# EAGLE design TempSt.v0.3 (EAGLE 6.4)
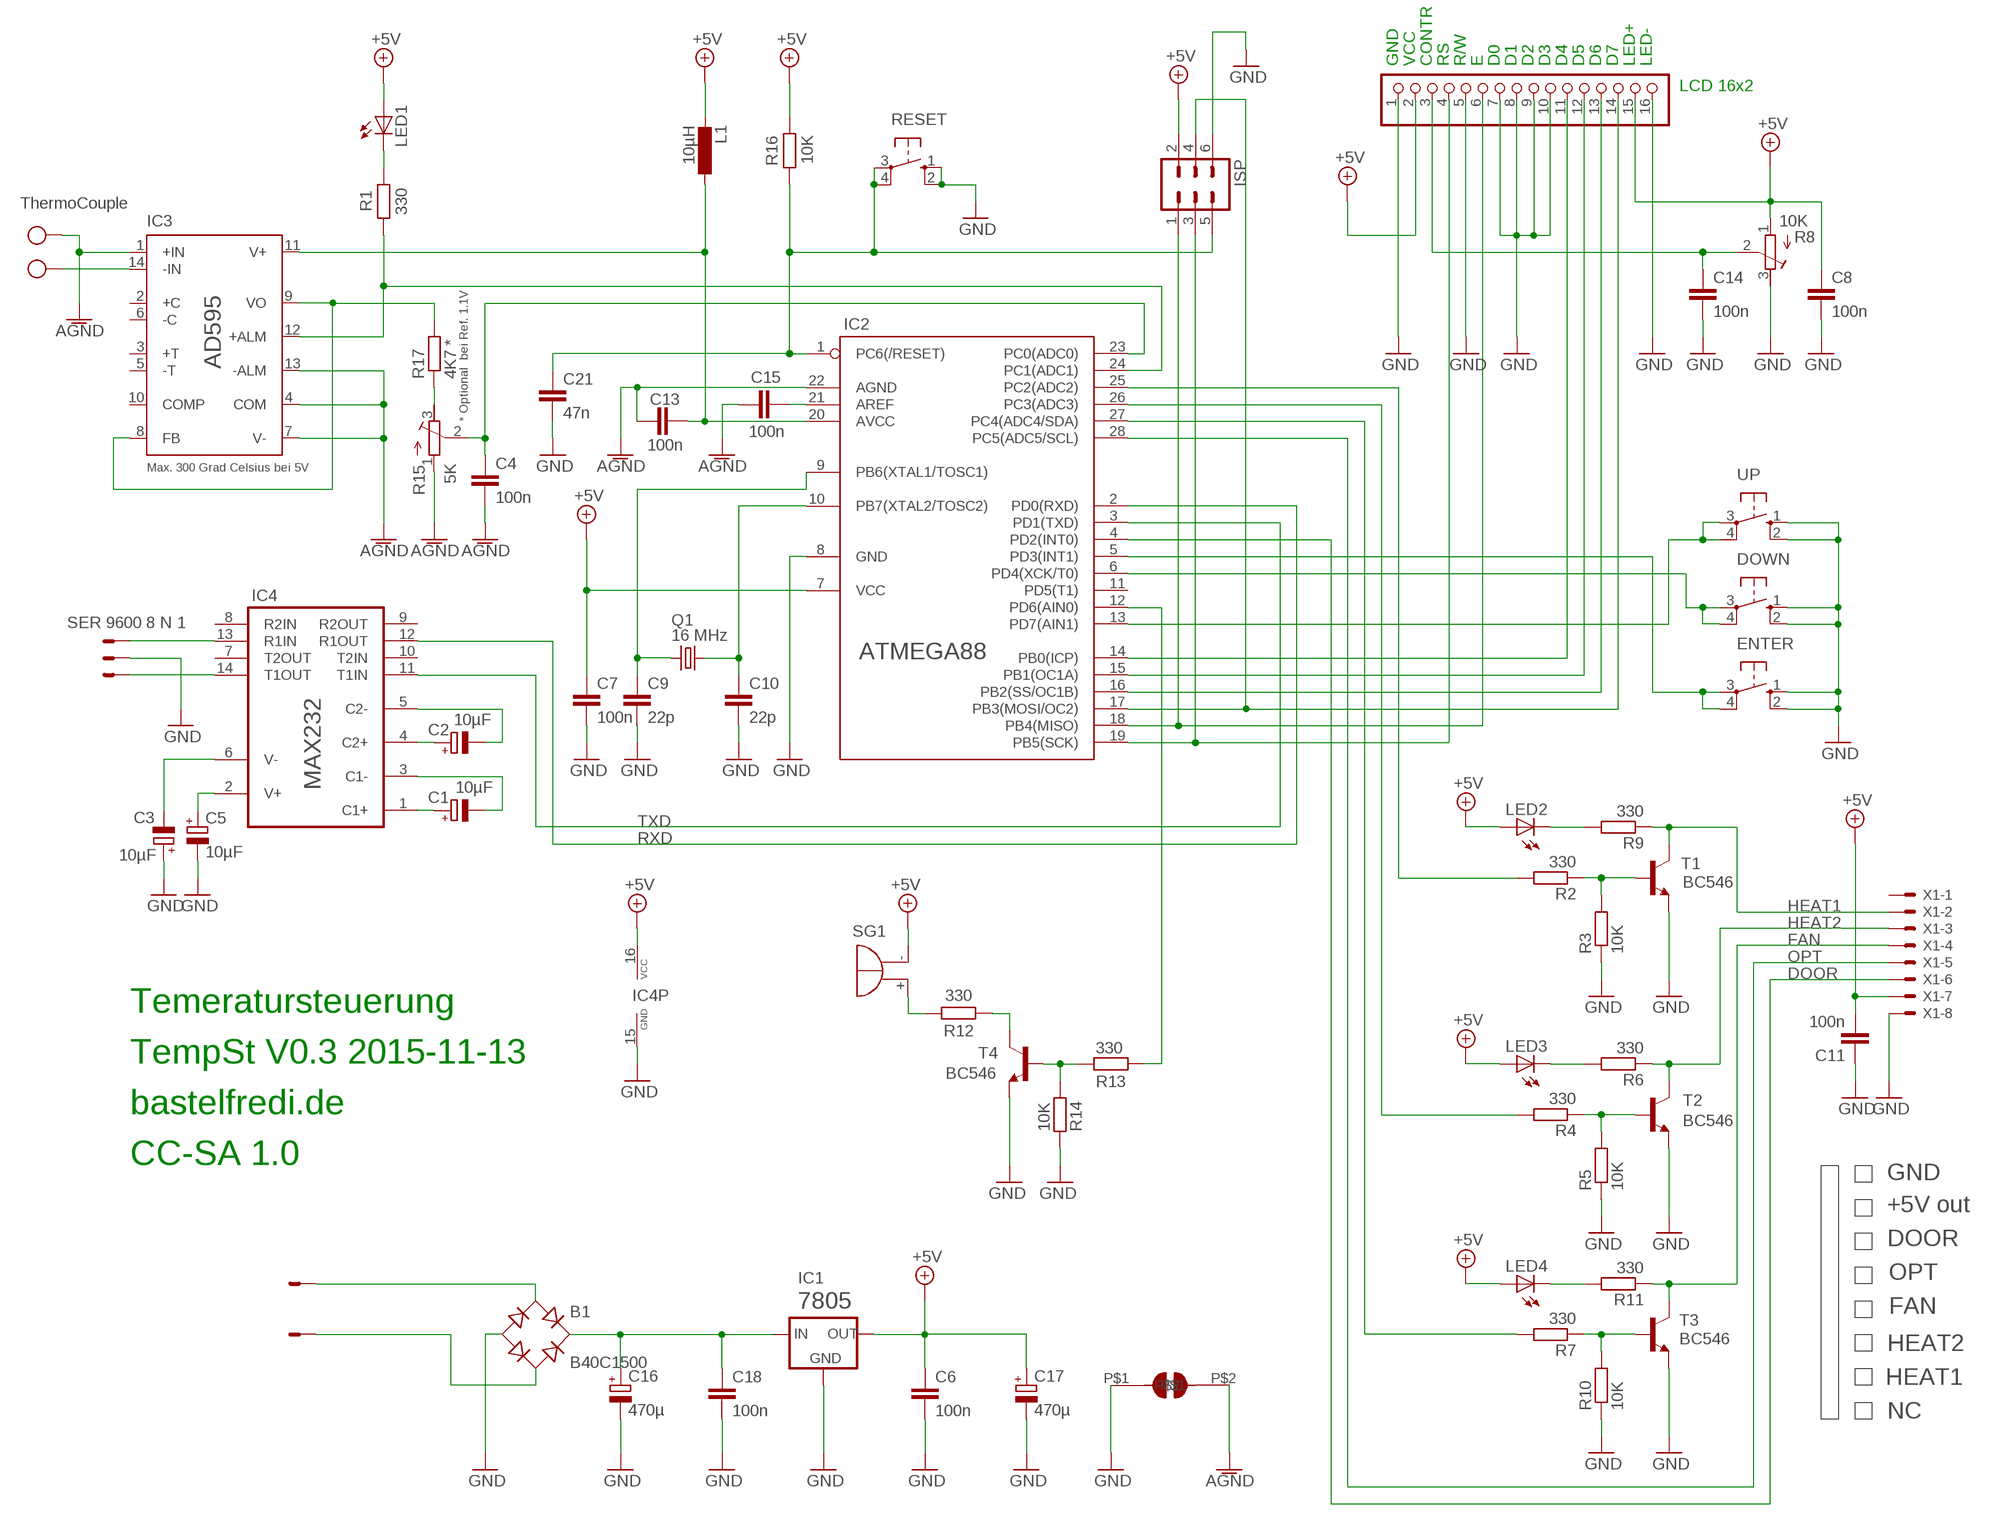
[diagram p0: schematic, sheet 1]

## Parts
B1  B40C1500  RB1A  [RB1A]
C1  10µF  CPOL-EUE2.5-6  [E2,5-6]
C2  10µF  CPOL-EUE2.5-6  [E2,5-6]
C3  10µF  CPOL-EUE2.5-6  [E2,5-6]
C4  100n  C-EU025-025X050  [C025-025X050]
C5  10µF  CPOL-EUE2.5-6  [E2,5-6]
C6  100n  C-EU050-035X075  [C050-035X075]
C7  100n  C-EU025-025X050  [C025-025X050]
C8  100n  C-EU025-025X050  [C025-025X050]
C9  22p  C-EU025-025X050  [C025-025X050]
C10  22p  C-EU025-025X050  [C025-025X050]
C11  100n  C-EU025-025X050  [C025-025X050]
C13  100n  C-EU025-025X050  [C025-025X050]
C14  100n  C-EU025-025X050  [C025-025X050]
C15  100n  C-EU025-025X050  [C025-025X050]
C16  470µ  CPOL-EUE5-10.5  [E5-10,5]
C17  470µ  CPOL-EUE5-10.5  [E5-10,5]
C18  100n  C-EU050-035X075  [C050-035X075]
C21  47n  C-EU050-025X075  [C050-025X075]
DOWN  10-XX  [B3F-10XX]
ENTER  10-XX  [B3F-10XX]
IC1  7805  78XXL  [78XXL]
IC2  ATMEGA88  MEGA8-P  [DIL28-3]
IC3  AD595  [DIL14]
IC4  MAX232  [DIL16]
ISP  ML6  [ML6]
JP3  LCD  PINHD-1X16  [1X16]
L1  10µH  L-EU0207/10  [0207/10]
LED1  LED3MM  [LED3MM]
LED2  LED3MM  [LED3MM]
LED3  LED3MM  [LED3MM]
LED4  LED3MM  [LED3MM]
Q1  16 MHz  CRYSTALHC49U-V  [HC49U-V]
R1  330  R-EU_0207/7  [0207/7]
R2  330  R-EU_0207/7  [0207/7]
R3  10K  R-EU_0207/7  [0207/7]
R4  330  R-EU_0207/7  [0207/7]
R5  10K  R-EU_0207/7  [0207/7]
R6  330  R-EU_0207/7  [0207/7]
R7  330  R-EU_0207/7  [0207/7]
R8  10K  R-TRIMM3339P  [RTRIM3339P]
R9  330  R-EU_0207/7  [0207/7]
R10  10K  R-EU_0207/7  [0207/7]
R11  330  R-EU_0207/7  [0207/7]
R12  330  R-EU_0207/7  [0207/7]
R13  330  R-EU_0207/7  [0207/7]
R14  10K  R-EU_0207/7  [0207/7]
R15  5K  R-TRIMM64W  [RTRIM64W]
R16  10K  R-EU_0207/7  [0207/7]
R17  4K7 *  R-EU_0207/10  [0207/10]
RESET  10-XX  [B3F-10XX]
SER  SER 9600 8 N 1  22-23-2031  [22-23-2031]
SG1  F/QMBIII  [F/QMBIII]
T1  BC546  BC548-NPN-TO92-CBE  [TO92-CBE]
T2  BC546  BC548-NPN-TO92-CBE  [TO92-CBE]
T3  BC546  BC548-NPN-TO92-CBE  [TO92-CBE]
T4  BC546  BC548-NPN-TO92-CBE  [TO92-CBE]
TC  ThermoCouple  AK500/2  [AK500/2]
U$1  SOLDER_JUMPER  [SOLDER_JUMPER]
UP  10-XX  [B3F-10XX]
X1  22-23-2081  [22-23-2081]
X4  22-23-2021  [22-23-2021]

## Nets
+5V: C6.1 C7.1 C8.1 C11.2 C17.+ IC1.OUT IC2.7(VCC) IC4.16(VCC) ISP.2 JP3.2 JP3.15 L1.2 LED1.A LED2.A LED3.A LED4.A R8.1(E) R16.2 SG1.-(+) X1.7
AGND: C4.2 C13.1 C15.2 IC2.22(AGND) IC3.1(+IN) IC3.4(COM) IC3.7(V-) IC3.13(-ALM) R15.1(E) TC.2 U$1.P$2
DOOR: IC2.4(PD2(INT0)) X1.6
ENTER: DOWN.3(P) DOWN.4(P1) IC2.6(PD4(XCK/T0))
FAN: R11.1 T3.C X1.4
GND: B1.- C3.+ C5.- C6.2 C7.2 C8.2 C9.2 C10.2 C11.1 C14.2 C16.- C17.- C18.2 C21.2 DOWN.1(S) DOWN.2(S1) ENTER.1(S) ENTER.2(S1) IC1.GND IC2.8(GND) IC4.15(GND) ISP.6 JP3.1 JP3.5 JP3.7 JP3.8 JP3.9 JP3.10 JP3.16 R3.1 R5.1 R8.3(A) R10.1 R14.1 RESET.1(S) RESET.2(S1) SER.2 T1.E T2.E T3.E T4.E U$1.P$1 UP.1(S) UP.2(S1) X1.8
HEAT1: R9.1 T1.C X1.2
HEAT2: R6.1 T2.C X1.3
N$1: IC4.14(T1OUT) SER.1
N$2: IC2.13(PD7(AIN1)) UP.3(P) UP.4(P1)
N$3: C15.1 IC2.21(AREF)
N$4: IC3.8(FB) IC3.9(VO) R17.2
N$5: IC2.17(PB3(MOSI/OC2)) ISP.4 JP3.14
N$6: IC2.18(PB4(MISO)) ISP.1 JP3.6
N$8: R12.1 SG1.+(-)
N$9: IC2.19(PB5(SCK)) ISP.3 JP3.4
N$10: LED1.K(C) R1.2
N$11: IC2.14(PB0(ICP)) JP3.11
N$12: IC2.15(PB1(OC1A)) JP3.12
N$13: IC2.16(PB2(SS/OC1B)) JP3.13
N$14: C14.1 JP3.3 R8.2(S)
N$15: IC2.24(PC1(ADC1)) IC3.12(+ALM) R1.1
N$16: B1.AC2 X4.1
N$17: B1.+ C16.+ C18.1 IC1.IN
N$18: IC4.13(R1IN) SER.3
N$20: LED2.K(C) R9.2
N$21: C5.+ IC4.2(V+)
N$22: C3.- IC4.6(V-)
N$23: C2.- IC4.5(C2-)
N$24: C1.- IC4.3(C1-)
N$25: C10.1 IC2.10(PB7(XTAL2/TOSC2)) Q1.2
N$26: C9.1 IC2.9(PB6(XTAL1/TOSC1)) Q1.1
N$27: C1.+ IC4.1(C1+)
N$28: C2.+ IC4.4(C2+)
N$29: R15.3(A) R17.1
N$30: R2.1 R3.2 T1.B
N$31: C21.1 IC2.1(PC6(/RESET)) ISP.5 R16.1 RESET.3(P) RESET.4(P1)
N$32: LED3.K(C) R6.2
N$33: IC2.25(PC2(ADC2)) R2.2
N$34: C4.1 IC2.23(PC0(ADC0)) R15.2(S)
N$35: R4.1 R5.2 T2.B
N$36: IC2.26(PC3(ADC3)) R4.2
N$37: LED4.K(C) R11.2
N$38: C13.2 IC2.20(AVCC) IC3.11(V+) L1.1
N$39: R7.1 R10.2 T3.B
N$40: IC2.27(PC4(ADC4/SDA)) R7.2
N$41: R12.2 T4.C
N$43: IC3.14(-IN) TC.1
N$46: R13.1 R14.2 T4.B
N$47: ENTER.3(P) ENTER.4(P1) IC2.5(PD3(INT1))
N$48: IC2.12(PD6(AIN0)) R13.2
N$49: B1.AC1 X4.2
OPT: IC2.28(PC5(ADC5/SCL)) X1.5
RXD: IC2.2(PD0(RXD)) IC4.12(R1OUT)
TXD: IC2.3(PD1(TXD)) IC4.11(T1IN)
Unconnected: IC2.11(PD5(T1)) IC3.2(+C) IC3.3(+T) IC3.5(-T) IC3.6(-C) IC3.10(COMP) IC4.7(T2OUT) IC4.8(R2IN) IC4.9(R2OUT) IC4.10(T2IN) X1.1

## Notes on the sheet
- GND | VCC | CONTR | RS | R/W | E | D0 | D1 | D2 | D3 | D4 | D5 | D6 | D7 | LED+ | LED-
- LCD 16x2
- * Optional  bei Ref. 1.1V
- Max. 300 Grad Celsius bei 5V
- Temeratursteuerung
- TempSt V0.3 2015-11-13
- bastelfredi.de
- CC-SA 1.0
- GND
- +5V out
- DOOR
- OPT
- FAN
- HEAT2
- HEAT1
- NC

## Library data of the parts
B1 = rectifier:RB1A: RECTIFIER 1 A
C1-C3 C5 C16 C17 = rcl:CPOL-EU: POLARIZED CAPACITOR, European symbol
C4 C6-C11 C13-C15 C18 C21 = rcl:C-EU: CAPACITOR, European symbol
DOWN ENTER RESET UP = buttons:10-XX: OMRON SWITCH
IC1 = v-reg:78XXL: VOLTAGE REGULATOR
IC2 = atmel:MEGA8-P: MICROCONTROLLER 8 Kbytes FLASH, 1 kbytes SRAM, 512 bytes EEPROM, USART, 4-channel 10 bit ADC, 2-channel 8 bit ADC Pin compatible with Atmega48, ATMega88, ATMega168 Source: avr.lbr
IC3 = analog-devices:AD595: ANALOG DEVICES; MPN: AD595AQ; OC_FARNELL: 409194; OC_NEWARK: 06WX1596
IC4 = maxim:MAX232: RS232 TRANSEIVER; MF: MAXIM; MPN: MAX232ACPE+; OC_FARNELL: 9723773; OC_NEWARK: 68K4544
ISP = con-harting-ml:ML6: HARTING; OC_FARNELL: unknown; OC_NEWARK: unknown
JP3 = pinhead:PINHD-1X16: PIN HEADER
L1 = rcl:L-EU: INDUCTOR, European symbol
LED1-LED4 = led:LED: LED
Q1 = crystal:CRYSTAL: CRYSTAL
R1-R7 R9-R14 R16 R17 = rcl:R-EU_: RESISTOR, European symbol
R8 R15 = rcl:R-TRIMM: Trimm resistor
SER = con-molex:22-23-2031: .100" (2.54mm) Center Header - 3 Pin; MF: MOLEX; MPN: 22-23-2031; OC_FARNELL: 1462950; OC_NEWARK: 30C0862
SG1 = buzzer:F/QMBIII: BUZZER; OC_FARNELL: unknown; OC_NEWARK: unknown
T1-T4 = transistor:*-NPN-: NPN Transistror BF959 corrected 2008.03.06
TC = con-ptr500:AK500/2: CONNECTOR; OC_FARNELL: unknown; OC_NEWARK: unknown
U$1 = th:SOLDER_JUMPER
X1 = con-molex:22-23-2081: .100" (2.54mm) Center Header - 8 Pin; MF: MOLEX; MPN: 22-23-2081; OC_FARNELL: 1756826; OC_NEWARK: 01C7592
X4 = con-molex:22-23-2021: .100" (2.54mm) Center Header - 2 Pin; MF: MOLEX; MPN: 22-23-2021; OC_FARNELL: 1462926; OC_NEWARK: 25C3832

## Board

Size 92.38 x 83.82 mm. Coordinates in mm from the lower left corner, seen from the top.
Outline: 0,83.81 92.38,83.81 92.38,0 0,0 0,83.82
Copper layers (1*16): Top 0.035mm / dielectric 1.5mm / Bottom 0.035mm
Design rules "default": minimum track width 10mil, minimum drill 24mil, track to track 8mil, track to pad 8mil, pad to pad 8mil, via to via 8mil, smd to smd 8mil, copper to edge 40mil, drill to drill 8mil, minimum pad ring 10mil, minimum via ring 8mil, stop-mask expansion 4mil, vias tented up to drill 0mil, thermal gap 10mil

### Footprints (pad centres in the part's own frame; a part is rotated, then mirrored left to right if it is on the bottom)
RB1A = drill 1.016: + -2.54,2.54 | drill 1.016 octagon: - 2.54,-2.54; AC1 2.54,2.54; AC2 -2.54,-2.54
E2,5-6 = drill 0.813 pad 1.6: + -1.27,0 | drill 0.813 pad 1.6 octagon: - 1.27,0
C025-025X050 = drill 0.813 octagon: 1 -1.27,0; 2 1.27,0
C050-035X075 = drill 0.813 octagon: 1 -2.54,0; 2 2.54,0
E5-10,5 = drill 1.016 pad 2.54: + -2.54,0 | drill 1.016 pad 2.54 octagon: - 2.54,0
C050-025X075 = drill 0.813 octagon: 1 -2.54,0; 2 2.54,0
B3F-10XX = drill 1.016 long: 1 -3.251,2.261; 2 3.251,2.261; 3 -3.251,-2.261; 4 3.251,-2.261
78XXL = drill 1.016 long: GND 0,-3.81; IN -2.54,-3.81; OUT 2.54,-3.81 | hole 3.302: 0,11.176
DIL28-3 = drill 0.813 long: 1 -16.51,-3.81; 2 -13.97,-3.81; 3 -11.43,-3.81; 4 -8.89,-3.81; 5 -6.35,-3.81; 6 -3.81,-3.81; 7 -1.27,-3.81; 8 1.27,-3.81; 9 3.81,-3.81; 10 6.35,-3.81; 11 8.89,-3.81; 12 11.43,-3.81; 13 13.97,-3.81; 14 16.51,-3.81; 15 16.51,3.81; 16 13.97,3.81; 17 11.43,3.81; 18 8.89,3.81; 19 6.35,3.81; 20 3.81,3.81; 21 1.27,3.81; 22 -1.27,3.81; 23 -3.81,3.81; 24 -6.35,3.81; 25 -8.89,3.81; 26 -11.43,3.81; 27 -13.97,3.81; 28 -16.51,3.81
DIL14 = drill 0.813 long: 1 -7.62,-3.81; 2 -5.08,-3.81; 3 -2.54,-3.81; 4 0,-3.81; 5 2.54,-3.81; 6 5.08,-3.81; 7 7.62,-3.81; 8 7.62,3.81; 9 5.08,3.81; 10 2.54,3.81; 11 0,3.81; 12 -2.54,3.81; 13 -5.08,3.81; 14 -7.62,3.81
DIL16 = drill 0.813 long: 1 -8.89,-3.81; 2 -6.35,-3.81; 3 -3.81,-3.81; 4 -1.27,-3.81; 5 1.27,-3.81; 6 3.81,-3.81; 7 6.35,-3.81; 8 8.89,-3.81; 9 8.89,3.81; 10 6.35,3.81; 11 3.81,3.81; 12 1.27,3.81; 13 -1.27,3.81; 14 -3.81,3.81; 15 -6.35,3.81; 16 -8.89,3.81
ML6 = drill 0.914 octagon: 1 -2.54,-1.27; 2 -2.54,1.27; 3 0,-1.27; 4 0,1.27; 5 2.54,-1.27; 6 2.54,1.27
1X16 = drill 1.016 long: 1 -19.05,0; 2 -16.51,0; 3 -13.97,0; 4 -11.43,0; 5 -8.89,0; 6 -6.35,0; 7 -3.81,0; 8 -1.27,0; 9 1.27,0; 10 3.81,0; 11 6.35,0; 12 8.89,0; 13 11.43,0; 14 13.97,0; 15 16.51,0; 16 19.05,0
0207/10 = drill 0.813 octagon: 1 -5.08,0; 2 5.08,0
LED3MM = drill 0.813 octagon: A -1.27,0; K 1.27,0
HC49U-V = drill 0.813: 1 -2.413,0; 2 2.413,0
0207/7 = drill 0.813 octagon: 1 -3.81,0; 2 3.81,0
RTRIM3339P = drill 0.61: 1 -2.54,0; 2 0,-2.54; 3 2.54,0
RTRIM64W = drill 0.61: 1 1.27,-2.54; 2 1.27,0; 3 1.27,2.54
22-23-2031 = drill 1 long: 1 -2.54,0; 2 0,0; 3 2.54,0
F/QMBIII = drill 0.914 pad 2.159 octagon: + 3.251,0; - -3.251,0
TO92-CBE = drill 0.813 long: B 0,0; C -2.54,0; E 2.54,0
AK500/2 = drill 1.321 long: 1 -2.515,0; 2 2.515,0
SOLDER_JUMPER = drill 0.8 square: P$1 -1.905,0; P$2 1.905,0
22-23-2081 = drill 1 long: 1 -8.89,0; 2 -6.35,0; 3 -3.81,0; 4 -1.27,0; 5 1.27,0; 6 3.81,0; 7 6.35,0; 8 8.89,0
22-23-2021 = drill 1 long: 1 -1.27,0; 2 1.27,0

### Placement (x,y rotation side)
B1  19.05,15.24 90 top
C1  87.63,16.51 90 top
C2  87.63,22.86 90 top
C3  87.63,29.21 270 top
C4  58.42,42.55 180 top
C5  87.63,10.16 270 top
C6  10.15,19.07 180 top
C7  59.69,62.23 180 top
C8  53.34,76.2 90 top
C9  53.34,60.96 270 top
C10  48.26,60.96 270 top
C11  71.12,11.43 90 top
C13  27.94,13.34 90 top
C14  6.35,73.66 180 top
C15  54.61,39.37 270 top
C16  11.43,7.62 90 top
C17  20.32,26.67 90 top
C18  7.62,15.24 0 top
C21  77.47,57.15 90 top
DOWN  87.63,60.96 270 top
ENTER  87.63,49.53 270 top
IC1  8.89,27.94 0 top
IC2  55.88,49.52 180 top
IC3  35.56,19.05 90 top
IC4  78.74,20.32 90 top
ISP  26.67,38.1 180 top
JP3  29.21,77.47 0 top
L1  27.94,22.23 90 top
LED1  45.72,8.89 180 top
LED2  45.72,31.75 0 top
LED3  45.72,24.13 0 top
LED4  45.72,16.51 0 top
Q1  50.8,66.04 180 top
R1  38.1,31.11 0 top
R2  60.96,33.02 0 top
R3  52.07,34.29 0 top
R4  60.96,25.4 0 top
R5  52.07,26.67 0 top
R6  52.07,22.86 180 top
R7  60.96,17.78 0 top
R8  7.62,67.31 270 top
R9  52.07,30.48 180 top
R10  52.07,19.05 0 top
R11  52.07,15.24 180 top
R12  71.12,67.31 180 top
R13  71.12,72.39 180 top
R14  71.12,76.2 180 top
R15  60.96,38.1 270 top
R16  73.66,59.69 90 top
R17  40.64,35.56 180 top
RESET  87.63,38.1 270 top
SER  80.01,5.08 0 top
SG1  76.2,37.47 0 top
T1  60.96,29.21 0 top
T2  60.96,21.59 0 top
T3  60.96,13.97 0 top
T4  78.74,72.39 90 top
TC  35.56,5.08 0 top
U$1  27.94,6.35 90 top
UP  87.63,72.39 270 top
X1  60.96,5.08 0 top
X4  21.59,5.08 0 top

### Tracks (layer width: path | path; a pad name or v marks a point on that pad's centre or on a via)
+5V  (via drill 0.6 pad 1.42)
  Top 1.016: v39.37,68.58 v17.78,68.58 | v17.78,64.77 v17.78,33.02
  Top 1.27: v44.45,29.21 v27.94,29.21 | v48.26,10.16 v68.58,10.16 | v60.96,64.77 v60.96,74.93
  Bottom 0.61: IC2.7
  Bottom 1.016: SG1.- 72.39,36.91 72.39,20.32 69.85,17.78 69.85,12.7 | IC4.16 73.66,11.43 72.39,12.7 C11.2 69.85,12.7 | 69.85,12.7 69.85,11.43 v68.58,10.16
  Bottom 1.27: X1.7 67.31,8.89 v68.58,10.16
  Bottom 1.778: R16.2 60.96,63.5 | 60.96,63.5 C7.1 60.96,58.42 57.15,54.61 IC2.7 | 12.7,69.85 16.51,69.85 v17.78,68.58 v17.78,64.77 | IC2.7 | LED2.A v44.45,29.21 LED3.A LED4.A 44.45,12.7 46.99,10.16 | L1.2 27.94,27.94 | 27.94,27.94 v27.94,29.21 | v27.94,29.21 27.94,31.75 | 27.94,31.75 27.94,33.02 | 27.94,33.02 27.94,34.29 29.21,35.56 ISP.2 | 12.7,69.85 R8.1 | JP3.15 45.72,73.66 | 45.72,73.66 44.45,73.66 v39.37,68.58 | 45.72,73.66 52.07,73.66 C8.1 v60.96,74.93 | v48.26,10.16 46.99,10.16 | 46.99,10.16 LED1.A | 60.96,63.5 v60.96,64.77 | JP3.2 12.7,69.85 | IC1.OUT 12.7,24.13 | C6.1 11.43,20.32 IC1.OUT | IC1.OUT C17.+ 24.13,24.13 26.67,26.67 | 26.67,26.67 27.94,27.94 | v17.78,33.02 24.13,33.02 | 24.13,33.02 25.4,31.75 | 25.4,31.75 26.67,30.48 | 26.67,30.48 v27.94,29.21 | 24.13,33.02 27.94,33.02 | 25.4,31.75 27.94,31.75 | 26.67,30.48 26.67,26.67
AGND  (1 unrouted)
  Bottom 0.61: 35.56,13.97 38.1,11.43
  Bottom 1.27: 36.83,19.05 36.83,15.24 35.56,13.97 IC3.13 | IC3.4 36.83,19.05 | 36.83,19.05 36.83,26.04 37.47,26.67 IC3.7 39.37,31.75 40.64,33.02 41.91,33.02 43.18,34.29 43.18,36.83 44.45,38.1 C15.2 57.15,38.1 | 57.15,41.91 IC2.22 | 57.15,41.91 57.15,39.37 57.15,38.1 | 30.48,13.97 28.57,12.06 C13.1 U$1.P$2 | 57.15,41.91 C4.2 | R15.1 57.15,38.1
  Bottom 1.778: IC3.1 39.37,6.38 TC.2 | IC3.1 38.1,10.16 38.1,5.08 36.83,6.35 | 36.83,6.35 36.83,10.16 38.1,11.43 IC3.1 | 36.83,6.35 36.83,5.08 38.1,3.81 39.37,5.08 39.37,6.35
DOOR
  Bottom 0.61: IC2.4 64.77,50.8 67.31,48.26 73.66,48.26 74.3,47.62 74.3,43.81 70.48,40.01 70.48,20.95 68.58,19.05 68.58,13.34 64.77,9.53 X1.6
ENTER
  Bottom 0.61: IC2.6 59.69,54.61 62.23,57.15 64.77,57.15 68.58,60.96 74.93,60.96 76.2,62.23 80.01,62.23 85.09,57.15 85.37,57.43 DOWN.4 DOWN.3
FAN
  Bottom 0.61: X1.4 59.69,10.16 58.42,11.43 T3.C 57.15,15.24 R11.1
GND  (via drill 0.6 pad 1.42, 0.8, 2)  (1 unrouted)
  Top 1.27: v58.42,78.74 v58.42,67.31 | v65.41,15.24 v71.75,15.24
  Bottom 0.61: 50.8,59.69 50.8,51.44 51.44,50.8 53.98,50.8 54.61,51.43 IC2.8 | R14.1 77.47,76.2 T4.E
  Bottom 1.016: C9.2 50.8,59.69 | 50.8,59.69 C10.2 | 57.15,62.23 57.15,57.78 54.61,55.24 IC2.8 | C21.2 79.38,59.69 83.82,55.24 89.89,55.24 | 50.8,59.69 50.8,67.31 52.07,68.58 55.88,68.58 57.15,67.31 57.15,62.23 | 57.15,62.23 C7.2 | 71.12,8.89 76.2,8.89 77.47,10.16 77.47,12.7 76.2,13.97 IC4.15 73.66,13.97 72.39,15.24 v71.75,15.24 | C3.+ 89.53,30.48 90.81,29.21 90.81,10.16 89.53,8.89 C5.- | T4.E 81.28,74.93 82.55,73.66 82.55,67.31 83.19,66.67 89.89,66.67 | X1.8 71.12,6.35 71.12,8.89 | 71.12,8.89 C11.1
  Bottom 1.27: JP3.7 25.4,81.28 | T3.E 63.5,15.24 | 63.5,15.24 62.23,16.51 62.23,19.05 63.5,20.32 T2.E 63.5,22.86 62.23,24.13 62.23,26.67 63.5,27.94 T1.E | R3.1 49.53,34.29 50.8,33.02 50.8,26.67 | R5.1 50.8,26.67 | 50.8,26.67 50.8,21.59 R10.1 50.8,16.51 50.8,8.26 49.53,6.99 49.53,1.27 | X1.8 69.85,1.27 | SER.2 80.01,1.27 | 33.02,81.28 JP3.10 | JP3.5 20.32,81.28 | JP3.8 27.94,81.28 | JP3.9 30.48,81.28 | 57.15,67.31 v58.42,67.31 | U$1.P$1 27.94,1.27 | v65.41,15.24 63.5,15.24
  Bottom 1.778: 48.26,81.28 33.02,81.28 30.48,81.28 27.94,81.28 25.4,81.28 20.32,81.28 11.43,81.28 10.16,80.01 JP3.1 6.35,77.47 2.54,73.66 | 48.26,81.28 JP3.16 C8.2 | v45.09,1.27 27.94,1.27 10.16,1.27 2.54,8.89 2.54,27.94 | v45.09,1.27 49.53,1.27 69.85,1.27 80.01,1.27 83.82,1.27 85.09,2.54 85.09,6.35 C5.- | 2.54,29.21 2.54,41.91 6.35,41.91 | 6.35,41.91 8.89,41.91 | 8.89,41.91 8.89,43.18 | 8.89,43.18 8.89,44.45 | 8.89,44.45 8.89,49.53 | 8.89,49.53 8.89,52.07 6.35,52.07 | 6.35,52.07 2.54,52.07 2.54,64.77 | 2.54,64.77 2.54,73.66 | 48.26,81.28 58.42,81.28 | 58.42,81.28 83.82,81.28 89.46,75.64 UP.1 UP.2 89.89,66.67 DOWN.1 DOWN.2 89.89,55.24 ENTER.1 ENTER.2 RESET.1 RESET.2 89.89,32.74 C3.+ | 2.54,64.77 R8.3 8.89,63.5 | C14.2 2.54,73.66 | 58.42,81.28 v58.42,78.74 | 8.89,27.94 10.16,29.21 13.97,29.21 | 8.89,27.94 IC1.GND 8.89,20.35 C6.2 10.16,16.51 C18.2 10.16,11.43 C16.- 12.7,11.43 12.7,12.7 15.24,15.24 19.05,15.24 B1.- | C17.- 15.24,29.21 | 15.24,29.21 13.97,29.21 | 2.54,27.94 2.54,29.21 | 2.54,29.21 3.81,29.21 | 3.81,29.21 7.62,29.21 8.89,27.94 | v45.09,5.08 v45.09,1.27 | ISP.6 15.24,36.83 | 15.24,36.83 13.97,36.83 | 13.97,36.83 13.97,35.56 | 13.97,35.56 13.97,30.48 | 13.97,30.48 13.97,29.21 | 8.89,41.91 13.97,41.91 13.97,38.1 | 13.97,38.1 13.97,36.83 | 6.35,52.07 8.89,49.53 | 6.35,41.91 8.89,44.45 | 8.89,43.18 11.43,43.18 11.43,41.91 12.7,40.64 12.7,36.83 10.16,34.29 8.89,34.29 5.08,38.1 5.08,40.64 11.43,40.64 11.43,36.83 10.16,35.56 8.89,35.56 6.35,38.1 6.35,39.37 10.16,39.37 10.16,38.1 | 10.16,38.1 10.16,36.83 8.89,36.83 7.62,38.1 10.16,38.1 | 15.24,36.83 13.97,35.56 | 15.24,29.21 13.97,30.48 | 15.24,36.83 13.97,38.1
  Bottom 1.778: 2.54,27.94 3.81,29.21
  other vias: 8.89,39.37
  pour Bottom (isolate 0.61): 44.45,69.22 56.52,69.22 58.42,67.31 58.42,55.88 57.15,54.61 46.99,54.61 44.45,57.15
  pour Bottom: 2.54,41.91 13.97,41.91 13.97,29.21 2.54,29.21
  pour Bottom: 8.89,41.91 13.97,41.91 13.97,57.15 13.97,58.42 7.62,64.77 2.54,64.77 2.54,52.07 8.89,52.07
HEAT1
  Bottom 0.61: T1.C 57.15,30.48 R9.1 53.34,27.94 53.34,21.59 52.7,20.95 52.7,12.06 54.61,10.16 X1.2
HEAT2
  Bottom 0.61: T2.C 57.15,22.86 R6.1 54.61,21.59 54.61,20.32 53.98,19.68 53.98,13.34 57.15,10.16 X1.3
N$1
  Bottom 0.61: SER.1 77.47,6.99 78.74,8.26 78.74,15.24 77.47,16.51 IC4.14
N$2
  Bottom 0.406: IC2.13
  Bottom 0.61: IC2.13 41.91,67.94 45.72,71.75 62.87,71.75 64.77,73.66 64.77,77.47 66.04,78.74 82.27,78.74 UP.3 UP.4
N$3
  Bottom 1.27: C15.1 IC2.21
N$4  (via drill 0.9 pad 1.68)
  Bottom 0.61: IC3.9 IC3.8 31.75,27.94 29.84,29.84 29.84,32.38 33.02,35.56 R17.2 v35.56,39.37
N$5  (via drill 0.6 pad 1.42)
  Top 0.61: v25.4,64.77 v39.37,64.77
  Bottom 0.406: IC2.17
  Bottom 0.61: JP3.14 43.18,76.2 36.83,69.85 36.83,67.31 v39.37,64.77 36.83,62.23 36.83,50.8 38.1,49.53 42.55,49.53 44.45,47.62 IC2.17 | ISP.4 27.94,38.1 27.94,43.18 25.4,45.72 v25.4,64.77
N$6  (via drill 0.6 pad 1.42)
  Top 0.61: v29.21,46.35 v33.66,46.35
  Bottom 0.61: IC2.18 46.99,44.45 45.72,43.18 36.83,43.18 v33.66,46.35 33.02,46.99 33.02,48.26 29.21,52.07 29.21,71.12 26.04,74.3 23.5,74.3 22.86,74.93 JP3.6 | ISP.1 v29.21,46.35
N$7  (via drill 2.2 pad 1.42)
  other vias: 90.17,81.28
N$8  (via drill 0.8 pad 1.42)
  Top 0.61: v83.19,62.23 v83.19,39.37
  Bottom 0.61: R12.1 78.11,67.31 v83.19,62.23 | v83.19,39.37 81.28,37.47 SG1.+
N$9
  Bottom 0.61: IC2.19 49.53,43.18 48.26,41.91 34.29,41.91 31.11,45.09 31.11,47.62 27.94,50.8 27.94,69.85 25.4,72.39 22.23,72.39 | 22.23,72.39 21.59,72.39 17.78,76.2 JP3.4 | ISP.3 26.67,41.27 23.5,44.45 23.5,60.96 22.23,62.23 22.23,72.39
N$10
  Bottom 0.61: LED1.K 41.91,11.43 R1.2
N$11  (via drill 0.6 pad 1.42)
  Top 0.61: v31.75,60.96 v39.37,60.96
  Bottom 0.406: IC2.14
  Bottom 0.61: JP3.11 35.56,76.2 31.75,72.39 v31.75,60.96 | v39.37,60.96 38.1,59.69 38.1,54.61 39.37,53.34 IC2.14
N$12
  Bottom 0.406: IC2.15
  Bottom 0.61: JP3.12 38.1,76.2 34.29,72.39 34.29,48.26 36.83,45.72 IC2.15
N$13
  Bottom 0.406: IC2.16
  Bottom 0.61: JP3.13 40.64,76.2 35.56,71.12 35.56,49.53 36.83,48.26 40.64,48.26 41.91,46.99 IC2.16
N$14
  Bottom 0.61: C14.1 5.08,71.12 R8.2 8.89,67.31 15.24,60.96 19.05,60.96 20.32,62.23 20.32,70.48 15.24,75.56 JP3.3
N$15
  Bottom 0.61: IC2.24 62.23,48.26 60.96,49.53 54.61,49.53 53.34,48.26 53.34,42.55 50.16,39.37 42.55,39.37 40,36.83 40.01,34.29 36.83,31.11 35.56,31.11 | R1.1 35.56,31.11 | 35.56,31.11 35.56,19.05 33.02,16.51 IC3.12
N$16
  Bottom 1.778: X4.1 20.32,11.43 B1.AC2
N$17
  Bottom 1.778: IC1.IN 5.08,22.86 C18.1 | C18.1 5.08,11.43 C16.+ 13.97,5.08 16.51,7.62 B1.+ | 5.08,16.51 C18.1
N$18
  Bottom 0.61: SER.3 82.55,7.62 80.01,10.16 80.01,16.51 77.47,19.05 IC4.13
N$20
  Bottom 0.61: R9.2 LED2.K
  Bottom 1.016: LED2.K 48.26,31.75 R9.2 46.99,30.48 LED2.K
N$21
  Bottom 0.61: IC4.2 83.82,13.97 86.36,16.51 88.9,16.51 89.53,15.88 89.53,13.34 C5.+
N$22
  Bottom 0.61: IC4.6 83.82,24.13 C3.-
N$23
  Bottom 0.61: IC4.5 83.82,21.59 86.36,24.13 C2.-
N$24
  Bottom 0.61: IC4.3 83.82,16.51 85.09,17.78 C1.-
N$25
  Bottom 0.61: IC2.10 49.53,55.88 48.26,57.15 46.99,57.15 45.72,58.42 45.72,60.96 46.99,62.23 C10.1 48.39,62.36 Q1.2
N$26
  Bottom 0.61: IC2.9 52.07,55.88 53.34,57.15 54.61,57.15 55.88,58.42 55.88,60.96 54.61,62.23 C9.1 53.21,62.36 Q1.1
N$27
  Bottom 0.61: IC4.1 83.82,11.43 C1.+
N$28
  Bottom 0.61: IC4.4 83.82,19.05 86.36,21.59 C2.+
N$29
  Bottom 0.61: R15.3 61.59,34.92 57.78,34.92 56.52,36.2 46.35,36.2 R17.1
N$30
  Bottom 0.61: T1.B 60.96,30.48 58.42,33.02 R2.1 R3.2
N$31  (via drill 0.6 pad 1.42)
  Top 0.61: v20.32,56.52 v71.12,56.52
  Bottom 0.61: 73.66,54.61 R16.1 73.03,56.52 v71.12,56.52 | 73.66,54.61 IC2.1 | 73.66,54.61 C21.1 79.38,54.61 84.45,49.53 86.36,49.53 87.63,48.26 87.63,43.61 RESET.3 RESET.4 | ISP.5 20.32,43.18 v20.32,56.52
N$32
  Bottom 0.61: R6.2 LED3.K
  Bottom 1.016: LED3.K 48.26,24.13 R6.2 46.99,22.86 LED3.K
N$33
  Bottom 0.61: IC2.25 64.77,44.45 65.41,43.81 65.41,33.66 R2.2
N$34
  Bottom 0.61: IC2.23 C4.1 59.69,40.64 60.96,39.37 R15.2
N$35
  Bottom 0.61: R5.2 R4.1 58.42,25.4 60.96,22.86 T2.B
N$36
  Bottom 0.61: IC2.26 67.31,44.45 66.67,43.81 66.67,36.2 66.67,27.3 R4.2
N$37
  Bottom 0.61: R11.2 LED4.K
  Bottom 1.016: LED4.K 48.26,16.51 R11.2 46.99,15.24 LED4.K
N$38
  Bottom 1.27: IC2.20 52.07,43.18 49.53,40.64 40.64,40.64 38.1,38.1 38.1,34.92 36.83,33.66 33.66,33.66 31.75,31.75 31.75,30.48 34.29,27.94 34.29,20.32 33.02,19.05 IC3.11 29.84,19.05 L1.1 C13.2
N$39
  Bottom 0.61: T3.B 60.96,15.24 58.42,17.78 R7.1 R10.2
N$40
  Bottom 0.406: IC2.27 69.85,45.72
  Bottom 0.61: 69.85,45.72 69.85,44.45 67.94,42.55 67.94,22.23 64.77,19.05 R7.2
N$41
  Bottom 0.61: R12.2 68.58,67.31 71.12,69.85 T4.C
N$43
  Bottom 1.778: 31.75,6.35 31.75,5.08 33.02,3.81 34.29,5.08 34.29,6.35 | IC3.14 31.75,6.38 TC.1 | IC3.14 33.02,10.16 33.02,5.08 34.29,6.35 | 34.29,6.35 34.29,10.16 33.02,11.43 IC3.14
N$44  (via drill 2.2 pad 1.42)
  other vias: 4.45,46.99
N$45  (via drill 2.2 pad 1.42)
  other vias: 79.38,46.99
N$46
  Bottom 0.61: R14.2 68.58,76.2 72.39,72.39 R13.1 T4.B
N$47  (1 unrouted)
  Bottom 0.61: IC2.5 62.23,54.61 63.5,55.88 67.31,55.88 69.85,58.42 74.93,58.42 76.83,56.52 80.01,56.52 83.74,52.78 ENTER.3
N$48
  Bottom 0.61: IC2.12 44.45,53.34 44.45,54.61 43.18,55.88 43.18,67.31 46.35,70.48 64.14,70.48 66.04,72.39 R13.2
N$49
  Bottom 1.778: X4.2 22.86,8.89 24.13,10.16 24.13,19.05 22.86,20.32 19.05,20.32 B1.AC1
N$50  (via drill 2.2 pad 1.42)
  other vias: 2.54,81.28
N$51  (via drill 2.2 pad 1.42)
  other vias: 2.54,2.54
N$52  (via drill 1 pad 2.18)
  other vias: 45.72,77.47
N$53  (via drill 2.2 pad 1.42)
  other vias: 90.17,2.54
OPT
  Bottom 0.61: IC2.28 72.39,44.45 69.21,41.27 69.22,21.59 67.31,19.68 67.31,13.97 62.23,8.89 X1.5
RXD
  Bottom 0.61: IC4.12 77.47,21.59 79.38,23.5 79.38,32.38 76.83,34.92 76.83,40.01 78.74,41.91 81.28,41.91 83.19,43.81 83.19,48.26 80.64,50.8 71.12,50.8 69.85,52.07 IC2.2
TXD
  Bottom 0.61: IC4.11 76.83,24.13 77.47,24.77 77.47,31.75 74.93,34.29 74.93,41.91 76.2,43.18 76.2,48.26 74.93,49.53 68.58,49.53 67.31,50.8 IC2.3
